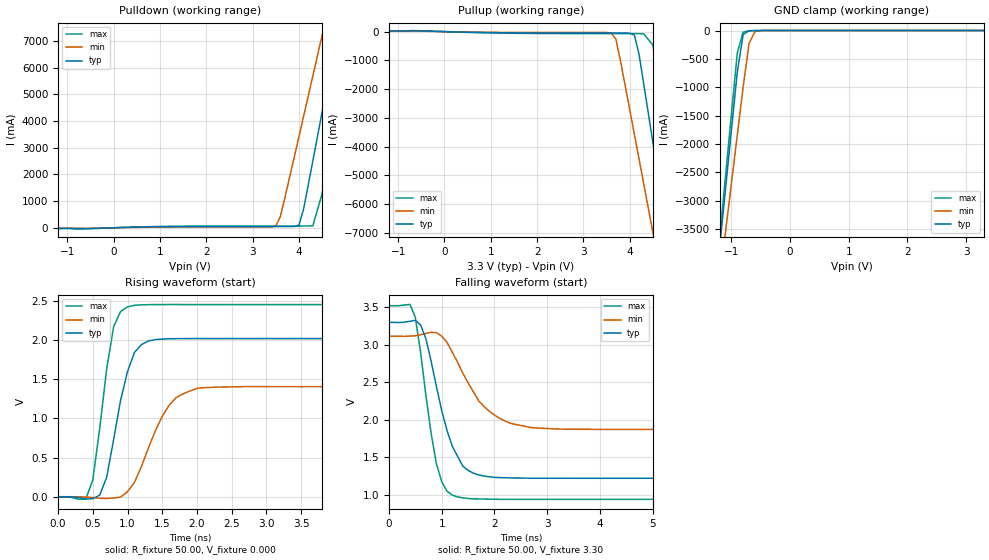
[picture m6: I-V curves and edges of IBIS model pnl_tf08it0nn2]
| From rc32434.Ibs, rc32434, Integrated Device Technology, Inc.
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[Model]   pnl_tf08it0nn2
Model_type   I/O
Polarity   Non-Inverting
Enable   Active-High
Vinl =  0.800V
Vinh =  2.000V
Vmeas =  1.500V
C_comp   0.40pF   0.30pF   0.50pF
[Temperature Range]   25.00   0.12k   0.000
[Voltage Range]   3.30V   3.00V   3.60V
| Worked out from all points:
|   slope of the pulldown table from 0 to 0.495 V, typ, clamps not added: 20.7 ohm
|   slope of the pullup table from 0 to 0.495 V, typ, clamps not added: 24.3 ohm
|   GND clamp passes 1 mA (typ) near -0.61 V on its own axis
|   rising waveform, R_fixture 50.00, V_fixture 0.000: 20-80 % time 275ps typ, 420ps min, 219ps max; typ from 0 V to 2.02 V
|   falling waveform, R_fixture 50.00, V_fixture 3.30: 20-80 % time 442ps typ, 666ps min, 312ps max; typ from 3.3 V to 1.22 V
[Pulldown]
| voltage   I(typ)   I(min)   I(max)
-3.3V     -30mA      -30mA      -30mA
3.5V      46.55mA    65.07mA    62.25mA
3.6V      46.65mA    425mA      62.38mA
4V        97.86mA    3.411A     63.28mA
4.1V      695mA      4.169A     64.13mA
4.3V      2.503A     5.688A     75.11mA
4.5V      4.333A     7.208A     1.27A
4.7V      6.168A     8.73A      3.2A
4.9V      8.006A     10.25A     5.141A
5.1V      9.846A     11.77A     7.086A
5.3V      11.68A     13.3A      9.034A
6.6V      23.67A     23.22A     21.73A
[Pullup]
| voltage   I(typ)   I(min)   I(max)
-3.3V     30mA       30mA       40mA
3.6V      -50.02mA   -51.55mA   -68.94mA
3.7V      -50.1mA    -260mA     -69.04mA
3.8V      -50.23mA   -1.024A    -69.14mA
4.1V      -121mA     -3.573A    -69.74mA
4.2V      -784mA     -4.428A    -71.35mA
4.3V      -1.805A    -5.284A    -75.13mA
4.5V      -3.869A    -6.999A    -468mA
4.7V      -5.941A    -8.716A    -2.627A
4.9V      -8.018A    -10.43A    -4.819A
5.1V      -10.09A    -12.15A    -7.019A
6.6V      -25.72A    -25.07A    -23.57A
[GND_clamp]
| voltage   I(typ)   I(min)   I(max)
-3.3V     -25.66A    -22.44A    -26.8A
-1.2V     -3.818A    -4.397A    -3.652A
-1.1V     -2.784A    -3.542A    -2.557A
-1V       -1.754A    -2.689A    -1.467A
-900mV    -733mA     -1.839A    -398mA
-800mV    -70.96mA   -994mA     -26.85mA
-700mV    -4.098mA   -230mA     -5.549mA
-600mV    -572uA     -20.8mA    -1.856mA
-400mV    -4.982uA   -63.15uA   -27.8uA
3.3V      168pA      102uA      -277pA
[Ramp]
| variable   typ   min   max
dV/dt_r   1.21/0.27n   0.84/0.42n   1.47/0.22n
dV/dt_f   1.25/0.44n   0.84/0.68n   1.52/0.34n
R_load = 50.00
[Rising Waveform]
R_fixture = 50.00
V_fixture = 0.000
| time   V(typ)   V(min)   V(max)
0s        0V         0V         0V
400ps     -28.88mV   -3.926mV   -29.01mV
500ps     -25.18mV   -10.46mV   212mV
700ps     247mV      -22.86mV   1.632V
800ps     731mV      -15.61mV   2.172V
1ns       1.599V     64.2mV     2.426V
1.2ns     1.943V     384mV      2.452V
1.6ns     2.018V     1.169V     2.456V
2ns       2.021V     1.385V     2.455V
9.9ns     2.021V     1.407V     2.455V
[Falling Waveform]
R_fixture = 50.00
V_fixture = 3.30
| time   V(typ)   V(min)   V(max)
0s        3.3V       3.115V     3.523V
400ps     3.315V     3.117V     3.539V
500ps     3.328V     3.122V     3.371V
700ps     3.086V     3.152V     2.333V
900ps     2.444V     3.163V     1.414V
1.2ns     1.648V     2.902V     995mV
1.4ns     1.382V     2.624V     958mV
1.8ns     1.249V     2.178V     942mV
2.7ns     1.22V      1.895V     938mV
9.9ns     1.219V     1.872V     938mV
